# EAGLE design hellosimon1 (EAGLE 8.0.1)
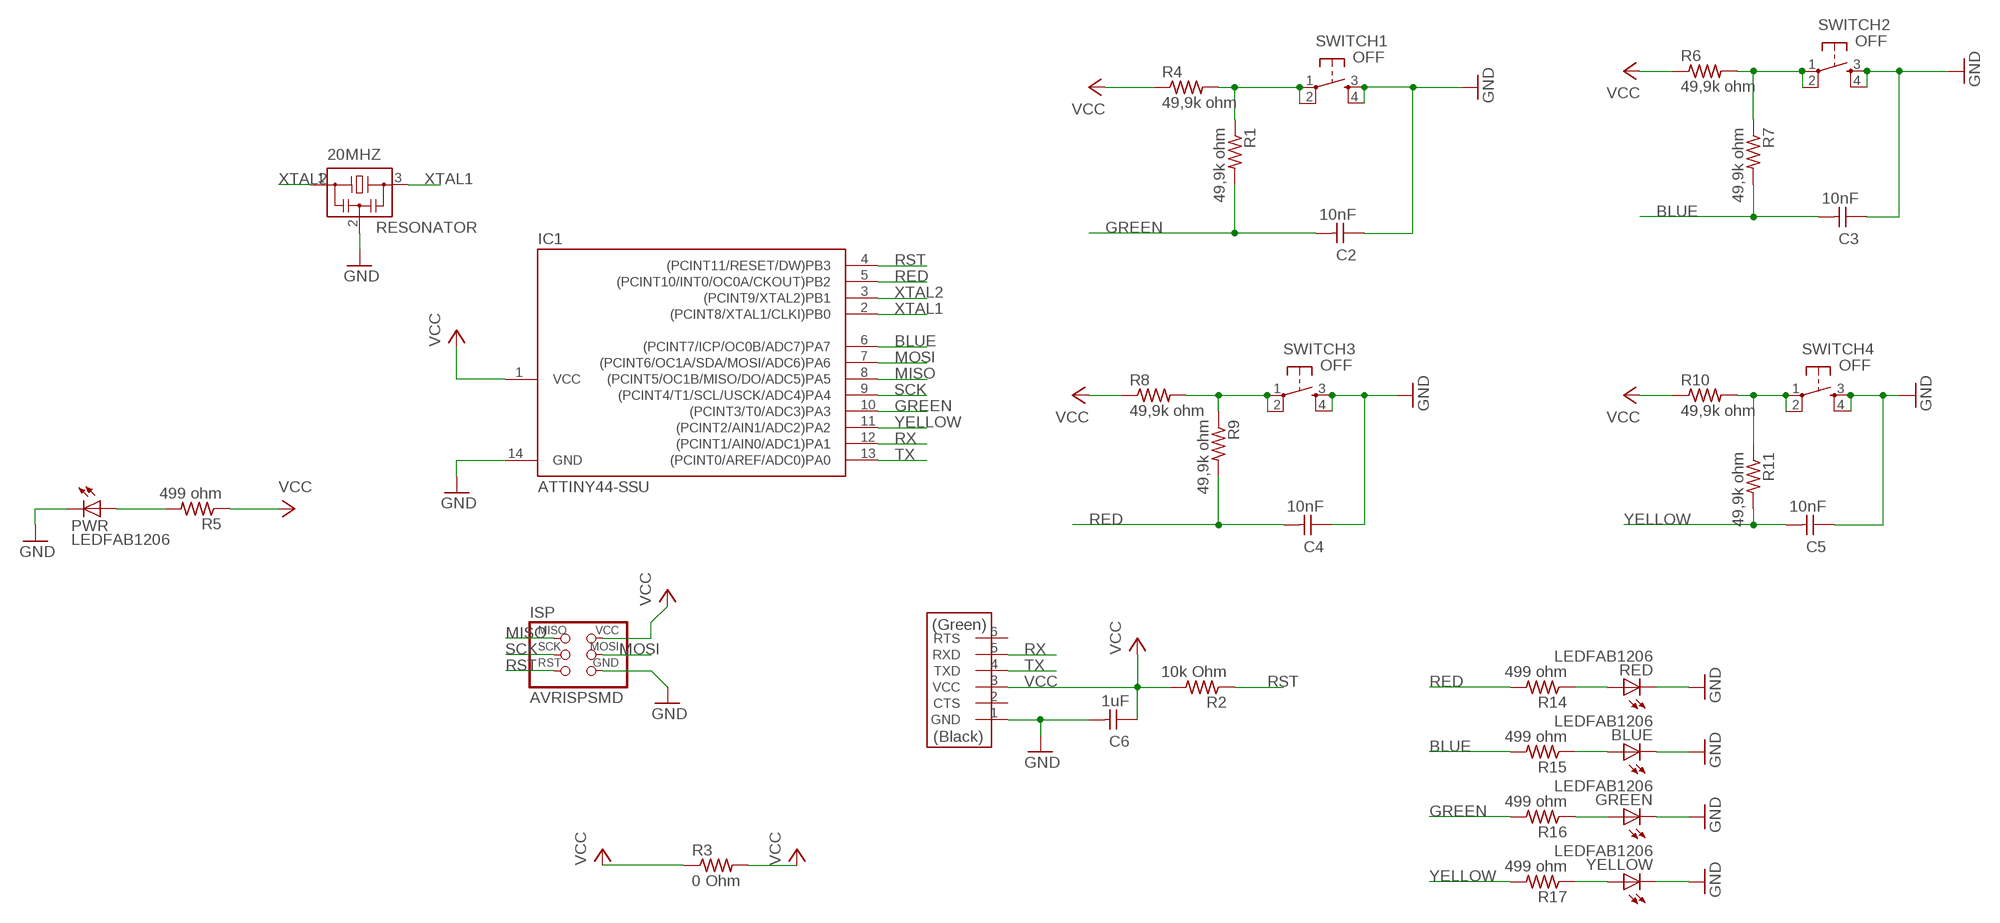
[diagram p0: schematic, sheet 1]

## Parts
20MHZ  RESONATOR  [EFOBM]
BLUE  LEDFAB1206  [LED1206FAB]
C2  10nF  CAP-UNPOLARIZEDFAB  [C1206FAB]
C3  10nF  CAP-UNPOLARIZEDFAB  [C1206FAB]
C4  10nF  CAP-UNPOLARIZEDFAB  [C1206FAB]
C5  10nF  CAP-UNPOLARIZEDFAB  [C1206FAB]
C6  1uF  CAP-UNPOLARIZEDFAB  [C1206FAB]
GREEN  LEDFAB1206  [LED1206FAB]
IC1  ATTINY44-SSU  [SOIC14]
ISP  AVRISPSMD  [2X03SMD]
PWR  LEDFAB1206  [LED1206FAB]
R1  49,9k ohm  RES-US1206FAB  [R1206FAB]
R2  10k Ohm  RES-US1206FAB  [R1206FAB]
R3  0 Ohm  RES-US1206FAB  [R1206FAB]
R4  49,9k ohm  RES-US1206FAB  [R1206FAB]
R5  499 ohm  RES-US1206FAB  [R1206FAB]
R6  49,9k ohm  RES-US1206FAB  [R1206FAB]
R7  49,9k ohm  RES-US1206FAB  [R1206FAB]
R8  49,9k ohm  RES-US1206FAB  [R1206FAB]
R9  49,9k ohm  RES-US1206FAB  [R1206FAB]
R10  49,9k ohm  RES-US1206FAB  [R1206FAB]
R11  49,9k ohm  RES-US1206FAB  [R1206FAB]
R14  499 ohm  RES-US1206FAB  [R1206FAB]
R15  499 ohm  RES-US1206FAB  [R1206FAB]
R16  499 ohm  RES-US1206FAB  [R1206FAB]
R17  499 ohm  RES-US1206FAB  [R1206FAB]
RED  LEDFAB1206  [LED1206FAB]
SWITCH1  OFF  6MM_SWITCH6MM_SWITCH  [6MM_SWITCH]
SWITCH2  OFF  6MM_SWITCH6MM_SWITCH  [6MM_SWITCH]
SWITCH3  OFF  6MM_SWITCH6MM_SWITCH  [6MM_SWITCH]
SWITCH4  OFF  6MM_SWITCH6MM_SWITCH  [6MM_SWITCH]
U$1  FTDI-SMD-HEADER  [1X06SMD]
YELLOW  LEDFAB1206  [LED1206FAB]

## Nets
BLUE: C3.2 IC1.6((PCINT7/ICP/OC0B/ADC7)PA7) R7.2 R15.2
GND: 20MHZ.2 BLUE.2(C) C2.1 C3.1 C4.1 C5.1 C6.2 GREEN.2(C) IC1.14(GND) ISP.6(GND) PWR.2(C) RED.2(C) SWITCH1.3(S) SWITCH1.4(S1) SWITCH2.3(S) SWITCH2.4(S1) SWITCH3.3(S) SWITCH3.4(S1) SWITCH4.3(S) SWITCH4.4(S1) U$1.1(GND) YELLOW.2(C)
GREEN: C2.2 IC1.10((PCINT3/T0/ADC3)PA3) R1.2 R16.2
MISO: IC1.8((PCINT5/OC1B/MISO/DO/ADC5)PA5) ISP.1(MISO)
MOSI: IC1.7((PCINT6/OC1A/SDA/MOSI/ADC6)PA6) ISP.4(MOSI)
N$1: R14.1 RED.1(A)
N$2: BLUE.1(A) R15.1
N$3: R1.1 R4.2 SWITCH1.1(P) SWITCH1.2(P1)
N$4: PWR.1(A) R5.2
N$5: GREEN.1(A) R16.1
N$6: R6.2 R7.1 SWITCH2.1(P) SWITCH2.2(P1)
N$7: R17.1 YELLOW.1(A)
N$10: R8.2 R9.1 SWITCH3.1(P) SWITCH3.2(P1)
N$13: R10.2 R11.1 SWITCH4.1(P) SWITCH4.2(P1)
RED: C4.2 IC1.5((PCINT10/INT0/OC0A/CKOUT)PB2) R9.2 R14.2
RST: IC1.4((PCINT11/RESET/DW)PB3) ISP.5(RST) R2.1
RX: IC1.12((PCINT1/AIN0/ADC1)PA1) U$1.5(RXD)
SCK: IC1.9((PCINT4/T1/SCL/USCK/ADC4)PA4) ISP.3(SCK)
TX: IC1.13((PCINT0/AREF/ADC0)PA0) U$1.4(TXD)
VCC: C6.1 IC1.1(VCC) ISP.2(VCC) R2.2 R3.1 R3.2 R4.1 R5.1 R6.1 R8.1 R10.1 U$1.3(VCC)
XTAL1: 20MHZ.3 IC1.2((PCINT8/XTAL1/CLKI)PB0)
XTAL2: 20MHZ.1 IC1.3((PCINT9/XTAL2)PB1)
YELLOW: C5.2 IC1.11((PCINT2/AIN1/ADC2)PA2) R11.2 R17.2
Unconnected: U$1.2(CTS) U$1.6(RTS)

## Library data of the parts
20MHZ = fab:RESONATOR
BLUE GREEN PWR RED YELLOW = fab:LED: LED
C2-C6 = fab:CAP-UNPOLARIZED
IC1 = fab:ATTINY44
ISP = fab:AVRISP
R1-R11 R14-R17 = fab:RES-US: Resistor (US Symbol)
SWITCH1-SWITCH4 = fab:6MM_SWITCH: OMRON SWITCH
U$1 = fab:FTDI-SMD-HEADER

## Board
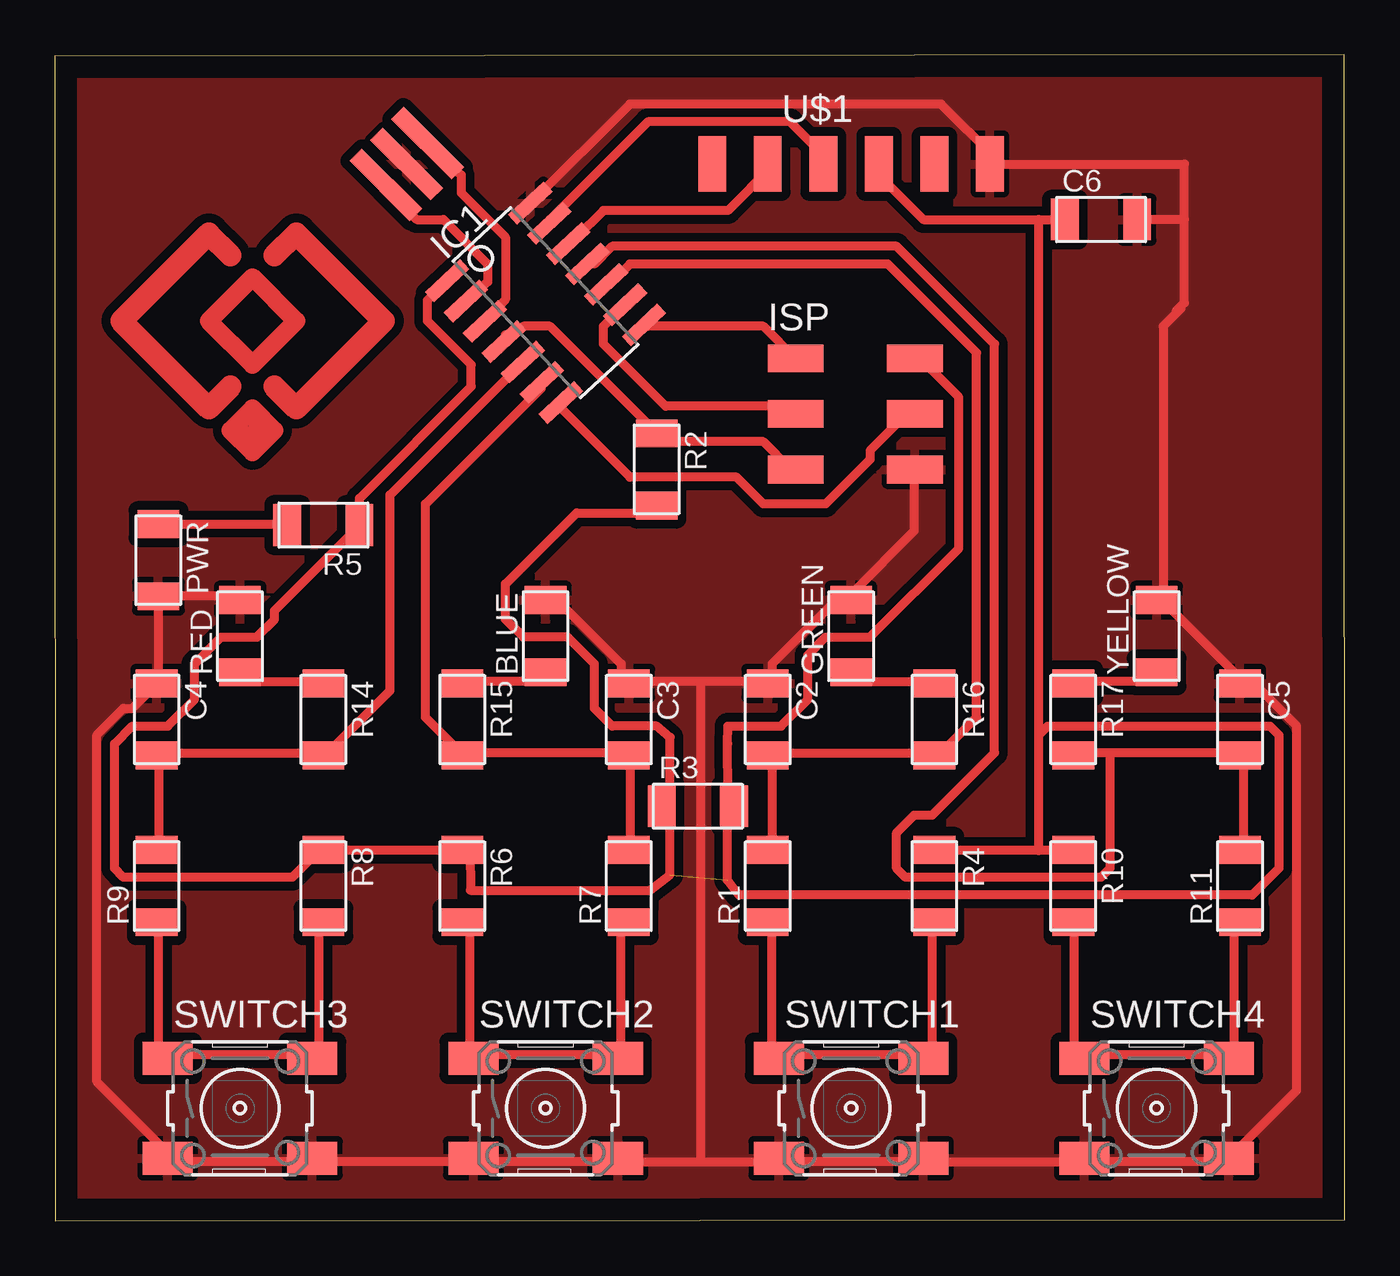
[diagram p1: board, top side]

Size 58.99 x 53.33 mm. Coordinates in mm from the lower left corner, seen from the top.
Outline: 0.03,0 58.99,0.06 58.96,53.33 0,53.27 0.03,0
Copper layers (1*16): Top 0.035mm / dielectric 1.5mm / Bottom 0.035mm
Design rules "hellosimon1": minimum track width 16mil, minimum drill 24mil, track to track 16mil, track to pad 16mil, pad to pad 0.205mm, via to via 0.205mm, smd to smd 8mil, copper to edge 40mil, drill to drill 8mil, minimum pad ring 10mil, minimum via ring 8mil, stop-mask expansion 4mil, vias tented up to drill 0mil, thermal gap 10mil

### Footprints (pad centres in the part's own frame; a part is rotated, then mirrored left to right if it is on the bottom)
EFOBM = smd 0.8 x 3.9: 1 -1.35,0; 2 0,0; 3 1.35,0
LED1206FAB = smd 1.27 x 1.905: 1 -1.651,0; 2 1.651,0
C1206FAB = smd 1.27 x 1.905: 1 -1.651,0; 2 1.651,0
SOIC14 = smd 0.61 x 2.21: 1 -3.81,-2.603; 2 -2.54,-2.603; 3 -1.27,-2.603; 4 0,-2.603; 5 1.27,-2.603; 6 2.54,-2.603; 7 3.81,-2.603; 8 3.81,2.603; 9 2.54,2.603; 10 1.27,2.603; 11 0,2.603; 12 -1.27,2.603; 13 -2.54,2.603; 14 -3.81,2.603
2X03SMD = smd 2.54 x 1.27: 1 -2.54,2.54; 2 2.92,2.54; 3 -2.54,0; 4 2.92,0; 5 -2.54,-2.54; 6 2.92,-2.54
R1206FAB = smd 1.27 x 1.905: 1 -1.651,0; 2 1.651,0
6MM_SWITCH = smd 2.286 x 1.524: 1 -3.302,2.286; 2 3.302,2.286; 3 -3.302,-2.286; 4 3.302,-2.286
1X06SMD = smd 2.54 x 1.27: 1 0,6.35; 2 0,3.81; 3 0,1.27; 4 0,-1.27; 5 0,-3.81; 6 0,-6.35

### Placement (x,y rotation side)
20MHZ  16.1,48.33 225 top
BLUE  22.45,26.74 90 top
C2  32.61,22.93 270 top
C3  26.26,22.93 270 top
C4  4.67,22.93 270 top
C5  54.2,22.93 270 top
C6  47.85,45.79 0 top
GREEN  36.42,26.74 90 top
IC1  22.45,41.98 313 top
ISP  36.42,36.9 0 top
PWR  4.74,30.22 270 top
R1  32.61,15.31 90 top
R2  27.53,34.36 270 top
R3  29.41,18.97 0 top
R4  40.23,15.31 270 top
R5  12.29,31.82 180 top
R6  18.64,15.31 270 top
R7  26.26,15.31 90 top
R8  12.29,15.31 270 top
R9  4.67,15.31 90 top
R10  46.58,15.31 270 top
R11  54.2,15.31 90 top
R14  12.29,22.93 270 top
R15  18.64,22.93 270 top
R16  40.23,22.93 270 top
R17  46.58,22.93 270 top
RED  8.48,26.74 90 top
SWITCH1  36.42,5.15 0 top
SWITCH2  22.45,5.15 0 top
SWITCH3  8.48,5.15 0 top
SWITCH4  50.39,5.15 0 top
U$1  36.42,48.33 270 top
YELLOW  50.39,26.74 90 top

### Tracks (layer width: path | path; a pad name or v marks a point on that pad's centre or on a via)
BLUE
  Top 0.406: R7.2 26.31,17.35 26.31,21 C3.2 25.9,21.41 18.99,21.41 R15.2 18.58,21.41 16.96,23.04 16.96,32.79 22.24,38.07 IC1.6
GND
  Top 0.406: 51.66,45.79 51.66,41.98 51.45,41.78 | 51.66,45.79 51.66,48.33 U$1.1 42.97,48.64 40.53,51.08 26.31,51.08 21.84,46.61 IC1.14 | 51.27,41.6 51.45,41.78 | 51.66,45.79 C6.2 | 51.45,41.78 51.5,41.73 50.69,40.92 50.69,28.72 YELLOW.2 50.69,28.32 54.35,24.66 C5.1 54.35,24.25 55.16,24.25 56.79,22.63 56.79,5.97 SWITCH4.4 53.54,2.72 47.44,2.72 SWITCH4.3 47.03,2.72 39.72,2.72 | 15.74,48.64 20MHZ.2 16.03,48.33 | BLUE.2 22.65,28.72 25.9,25.47 25.9,24.66 C3.1 26.31,24.66 29.56,24.66 | ISP.6 39.31,34.01 39.31,31.57 36.47,28.72 GREEN.2 36.06,28.72 32.81,25.47 32.81,24.66 C2.1 32.4,24.66 29.56,24.66 | 39.72,2.72 33.22,2.72 SWITCH1.3 32.81,2.72 29.56,2.72 | 29.56,2.72 25.9,2.72 SWITCH2.4 25.49,2.72 19.4,2.72 SWITCH2.3 18.99,2.72 12.08,2.72 SWITCH3.4 11.68,2.72 5.17,2.72 SWITCH3.3 5.17,3.12 1.92,6.37 1.92,22.22 3.14,23.44 3.55,23.44 4.36,24.25 C4.1 4.74,24.66 PWR.2 8.3,28.57 RED.2 | 39.72,2.72 SWITCH1.4 | 29.56,2.72 29.56,24.66
  pour Top (isolate 0.254): 0.05,53.15 0.05,0.15 59.05,0.15 59.05,53.15
GREEN
  Top 0.406: R1.2 32.81,17.35 32.81,21 C2.2 32.81,21.41 40.12,21.41 R16.2 40.53,21.41 42.16,23.04 42.16,39.7 38.09,43.76 26.31,43.76 25.49,42.95 IC1.10
MISO
  Top 0.406: ISP.1 32.4,40.92 27.12,40.92 IC1.8
MOSI
  Top 0.406: IC1.7 23.06,37.26 26.31,34.01 31.18,34.01 32.4,32.79 35.25,32.79 37.28,34.82 37.28,35.23 39.31,37.26 ISP.4
N$1
  Top 0.406: R14.1 12.08,24.66 9.24,24.66 8.83,25.07 RED.1
N$2
  Top 0.406: R15.1 18.99,24.66 21.84,24.66 22.24,25.07 BLUE.1
N$3
  Top 0.406: R1.1 32.81,13.28 32.81,7.59 SWITCH1.1 33.22,7.59 39.72,7.59 | 39.72,7.59 40.12,8 40.12,13.28 R4.2 | 39.72,7.59 SWITCH1.2
N$4
  Top 0.406: PWR.1 10.59,31.87 R5.2
N$5
  Top 0.406: R16.1 40.12,24.66 36.87,24.66 36.47,25.07 GREEN.1
N$6
  Top 0.406: R6.2 18.99,13.28 18.99,7.59 SWITCH2.1 19.4,7.59 25.49,7.59 SWITCH2.2 25.9,7.59 25.9,13.28 R7.1
N$7
  Top 0.406: R17.1 46.63,24.66 49.88,24.66 50.28,25.07 YELLOW.1
N$8
  Top 0.406: 9.05,37.15 9.05,35.15 | 8.05,36.15 10.05,36.15
  Top 0.813: 8.05,36.15 9.05,37.15 10.05,36.15 9.05,35.15 8.05,36.15
N$9
  Top 1.016: 8.05,38.15 7.05,37.15 3.05,41.15 7.05,45.15 8.05,44.15
N$10
  Top 0.406: 5.17,7.59 4.77,8 4.77,13.28 R9.1 | R8.2 12.08,13.28 12.08,7.59 SWITCH3.2 11.68,7.59 5.17,7.59 | 5.17,7.59 SWITCH3.1
N$11
  Top 0.813: 9.05,43.15 7.05,41.15 9.05,39.15 11.05,41.15 9.05,43.15
N$12
  Top 1.016: 10.05,44.15 11.05,45.15 15.05,41.15 11.05,37.15 10.05,38.15
N$13
  Top 0.406: R10.2 46.63,13.28 46.63,8 47.03,7.59 SWITCH4.1 47.44,7.59 53.54,7.59 SWITCH4.2 53.94,7.59 53.94,13.28 R11.1
RED
  Top 0.406: R9.2 4.77,17.35 4.77,21 C4.2 4.77,21.41 12.08,21.41 R14.2 12.49,21.41 15.33,24.25 15.33,33.2 21.02,38.88 IC1.5
RST
  Top 0.406: ISP.5 33.62,34.41 32.4,35.63 27.53,35.63 R2.1 27.53,36.04 22.65,40.92 21.43,40.92 21.02,40.51 20.62,40.51 IC1.4
RX
  Top 0.406: IC1.12 23.87,44.98 25.09,46.2 30.78,46.2 32.81,48.23 U$1.5
SCK
  Top 0.406: IC1.9 25.9,41.73 25.09,40.92 25.09,40.1 27.93,37.26 33.62,37.26 ISP.3
TX
  Top 0.406: IC1.13 22.65,45.79 27.12,50.26 33.62,50.26 35.25,48.64 U$1.4
VCC  (1 unrouted)
  Top 0.406: 45,45.79 39.72,45.79 37.69,47.83 U$1.3 | 45,45.79 C6.1 | 45,16.94 46.22,16.94 R10.1 | 45,16.94 40.53,16.94 R4.1 | 45,22.22 45.41,22.63 55.57,22.63 55.97,22.22 55.97,16.13 54.75,14.91 31.3,14.91 30.75,15.59 30.75,18.27 30.78,18.56 R3.2 30.78,19.57 30.77,21.82 30.78,22.63 33.22,22.63 34.43,23.85 34.43,25.88 35.25,26.69 37.28,26.69 41.34,30.76 41.34,37.67 39.72,39.29 ISP.2 | 45,16.94 45,22.22 | 45,22.22 45,45.79 | 18.99,16.94 19.01,15.12 27.23,15.12 28.13,15.83 28.13,18.79 R3.1 | R2.2 27.53,32.38 23.87,32.38 20.62,29.13 20.62,27.51 21.43,26.69 23.46,26.69 24.68,25.47 24.68,23.44 25.49,22.63 27.53,22.63 28.14,22.12 28.15,19.28 R3.1 | 27.93,18.56 R3.1 | 18.99,16.53 18.99,16.94 | 18.99,16.94 R6.1 18.58,16.94 12.49,16.94 R8.1 12.08,16.94 10.86,15.72 3.14,15.72 2.74,16.13 2.74,21.82 3.55,22.63 5.17,22.63 6.39,23.85 6.39,25.47 7.61,26.69 9.24,26.69 10.05,27.51 10.05,27.91 13.71,31.57 R5.1 13.94,33.04 19.05,38.15 19.05,39.15 17.05,41.15 17.05,42.1 IC1.1
XTAL1
  Top 0.406: IC1.2 18.99,42.14 19.8,42.95 19.8,43.76 17.77,45.79 16.55,45.79 15.33,47.01 20MHZ.3
XTAL2
  Top 0.406: IC1.3 19.8,41.32 20.62,42.14 20.62,44.98 18.58,47.01 18.58,47.83 17.37,49.04 20MHZ.1
YELLOW
  Top 0.406: R11.2 54.35,17.35 54.35,21 C5.2 53.94,21.41 48.25,21.41 | 48.25,21.41 46.63,21.41 R17.2 | 48.25,21.41 48.25,16.13 47.85,15.72 38.9,15.72 38.5,16.13 38.5,17.75 39.31,18.56 40.12,18.56 42.97,21.41 42.97,40.1 38.5,44.57 25.49,44.57 24.68,43.76 IC1.11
